FUNCTION_BLOCK FB_LN_IED_LD1_LEDGGIO4 EXTENDS FB_AcsiCommonLogicalNodeClass
VAR_INPUT
	NamPlt: FB_DO_IED_LD1_LEDGGIO4_NamPlt := (sClass:='LPL', bLinkResult:=THIS^.AddDataToContainer(ipData:=NamPlt));
	Beh: FB_DO_IED_LD1_LEDGGIO4_Beh := (sClass:='ENS', bLinkResult:=THIS^.AddDataToContainer(ipData:=Beh));
	Health: FB_DO_IED_LD1_LEDGGIO4_Health := (sClass:='ENS', bLinkResult:=THIS^.AddDataToContainer(ipData:=Health));
	Mod_: FB_DO_IED_LD1_LEDGGIO4_Mod := (sObjectName:='Mod', sClass:='ENC', bLinkResult:=THIS^.AddDataToContainer(ipData:=Mod_));
	AnOut1: FB_DO_IED_LD1_LEDGGIO4_AnOut1 := (sClass:='APC', bLinkResult:=THIS^.AddDataToContainer(ipData:=AnOut1));
	SPCSO1: FB_DO_IED_LD1_LEDGGIO4_SPCSO1 := (sClass:='SPC', bLinkResult:=THIS^.AddDataToContainer(ipData:=SPCSO1));
	DPCSO1: FB_DO_IED_LD1_LEDGGIO4_DPCSO1 := (sClass:='DPC', bLinkResult:=THIS^.AddDataToContainer(ipData:=DPCSO1));
	ISCSO1: FB_DO_IED_LD1_LEDGGIO4_ISCSO1 := (sClass:='INC', bLinkResult:=THIS^.AddDataToContainer(ipData:=ISCSO1));
END_VAR
VAR
END_VAR

END_FUNCTION_BLOCK
